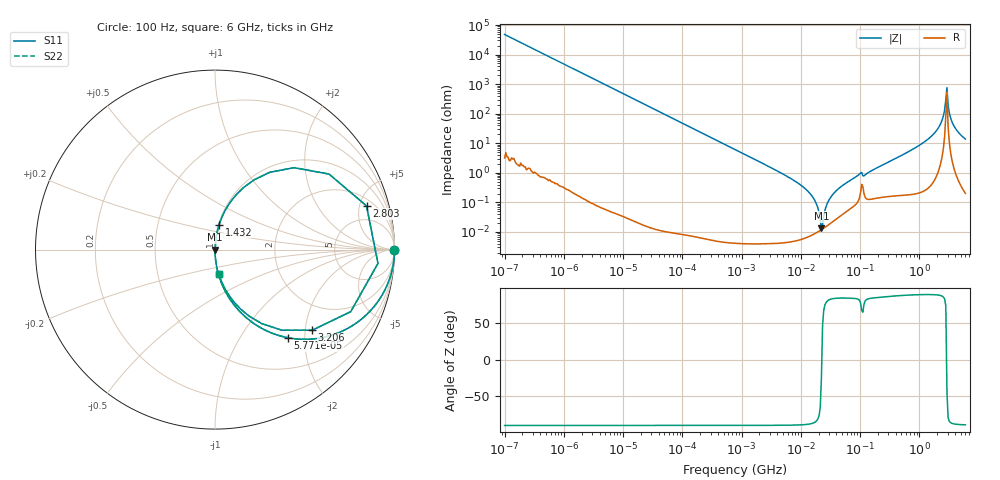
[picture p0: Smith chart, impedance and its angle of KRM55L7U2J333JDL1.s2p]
!Murata Part Number: KRM55L7U2J333JDL1
!These Parameters are Measured in Series Mode Connection
!Data Generated on Jan 08, 2026
!  o--ll--o
!Port1  Port2
!  o------o
!Operation Temp=25[degC], DC Bias Voltage=0[V]
!Freq. Start=100[Hz] Stop=6[GHz] 401[Steps]
# Hz S RI R 50
!Freq.(Hz) S11(Real) S11(Imag) S21(Real) S21(Imag) S12(Real) S12(Imag) S22(Real) S22(Imag)
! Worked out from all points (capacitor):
!   401 points, 100 Hz to 6 GHz, reference 50 ohm
!   read as one part in series: C = 33.2 nF near 109 Hz
!   lowest |Z| = 13.3 mohm at 22.26 MHz (marker M1)
!   series resonance near 22.58 MHz, so ESL is about 1.5 nH
!   S11 on the Smith chart (normalised r, x): 100 Hz: open; 57.71 kHz: 1.00, -1.66; 1.432 GHz: 1.01, +0.29; 2.803 GHz: 2.73, +5.83; 3.206 GHz: 1.22, -2.18; 6 GHz: 1.00, -0.28
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100  1 -0.00209  4.5e-06 0.00209  4.5e-06 0.00209  1 -0.00209
2008  0.9982 -0.0419  0.00176 0.0419  0.00176 0.0419  0.9982 -0.0419
13772  0.9236 -0.2655  0.0764 0.2655  0.0764 0.2655  0.9236 -0.2655
40335  0.5851 -0.4927  0.4149 0.4927  0.4149 0.4927  0.5851 -0.4927
57709  0.4079 -0.4914  0.5921 0.4914  0.5921 0.4914  0.4079 -0.4914
154540  0.0877 -0.2828  0.9123 0.2828  0.9123 0.2828  0.0877 -0.2828
774597  0.00384 -0.0615  0.9962 0.0615  0.9962 0.0615  0.00384 -0.0615
6948629  8.56e-05 -0.00624  0.9999 0.00624  0.9999 0.00624  8.56e-05 -0.00624
1.555665e7  8.15e-05 -0.00161  0.9999 0.00161  0.9999 0.00161  8.15e-05 -0.00161
2.225763e7  0.000119 -5.95e-05  0.9999 5.95e-05  0.9999 5.95e-05  0.000119 -5.95e-05
2.434276e7  0.000134 0.000318  0.9999 -0.000318  0.9999 -0.000318  0.000134 0.000318
3.045065e7  0.000186 0.00127  0.9998 -0.00127  0.9998 -0.00127  0.000186 0.00127
4.35672e7  0.000323 0.00293  0.9997 -0.00293  0.9997 -0.00293  0.000323 0.00293
9.753859e7  0.00149 0.00891  0.9985 -0.00891  0.9985 -0.00891  0.00149 0.00891
3.124326e8  0.00216 0.0238  0.9978 -0.0238  0.9978 -0.0238  0.00216 0.0238
1.431855e9  0.0228 0.1389  0.9772 -0.1389  0.9772 -0.1389  0.0228 0.1389
2.240541e9  0.1594 0.346  0.8406 -0.346  0.8406 -0.346  0.1594 0.346
2.562649e9  0.4405 0.4565  0.5595 -0.4565  0.5595 -0.4565  0.4405 0.4565
2.802721e9  0.8442 0.2435  0.1558 -0.2435  0.1558 -0.2435  0.8442 0.2435
3.205649e9  0.5409 -0.4494  0.4591 0.4494  0.4591 0.4494  0.5409 -0.4494
3.8344e9  0.1407 -0.3295  0.8593 0.3295  0.8593 0.3295  0.1407 -0.3295
6e9  0.0209 -0.1359  0.9791 0.1359  0.9791 0.1359  0.0209 -0.1359
